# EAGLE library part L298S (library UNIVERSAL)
L298 pre SMD montaz.
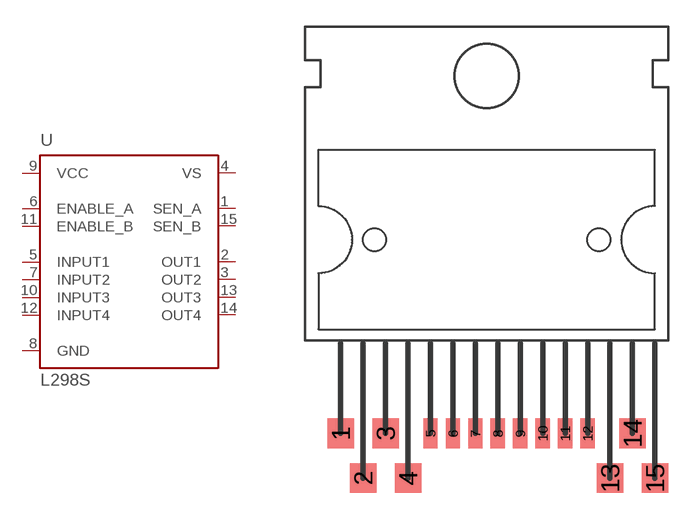
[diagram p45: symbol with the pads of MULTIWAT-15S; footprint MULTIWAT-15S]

Designator prefix -

## L298S  [MULTIWAT-15S]
1  SEN_A  in
2  OUT1  out
3  OUT2  out
4  VS  pwr
5  INPUT1  in
6  ENABLE_A  in
7  INPUT2  in
8  GND  pwr
9  VCC  pwr
10  INPUT3  in
11  ENABLE_B  in
12  INPUT4  in
13  OUT3  out
14  OUT4  out
15  SEN_B  in

## Footprint MULTIWAT-15S (pad centres in mm)
smd 1.5 x 1.676: 1 -8.89,0; 2 -7.62,-2.54; 3 -6.35,0; 4 -5.08,-2.54; 13 6.35,-2.54; 14 7.62,0; 15 8.89,-2.54
smd 0.813 x 1.676: 5 -3.81,0; 6 -2.54,0; 7 -1.27,0; 8 0,0; 9 1.27,0; 10 2.54,0; 11 3.81,0; 12 5.08,0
